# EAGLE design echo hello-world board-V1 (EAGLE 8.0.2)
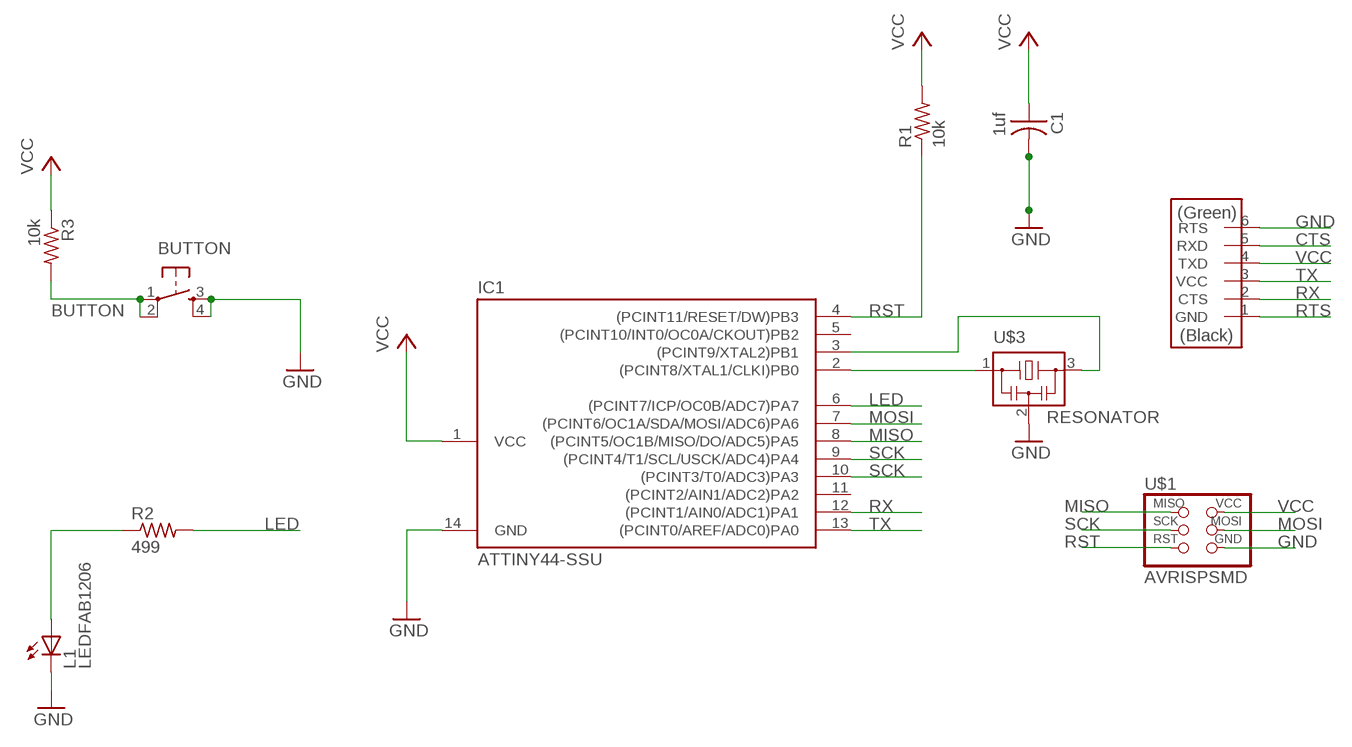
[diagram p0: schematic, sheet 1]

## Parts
BUTTON  6MM_SWITCH6MM_SWITCH  [6MM_SWITCH]
C1  1uf  CAP-US1206FAB  [C1206FAB]
IC1  ATTINY44-SSU  [SOIC14]
L1  LEDFAB1206  [LED1206FAB]
R1  10k  RES-US1206FAB  [R1206FAB]
R2  499  RES-US1206FAB  [R1206FAB]
R3  10k  RES-US1206FAB  [R1206FAB]
U$1  AVRISPSMD  [2X03SMD]
U$2  FTDI-SMD-HEADER  [1X06SMD]
U$3  RESONATOR  [EFOBM]

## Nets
BUTTON: BUTTON.1(P) BUTTON.2(P1) IC1.10((PCINT3/T0/ADC3)PA3) R3.2
CTS: U$2.5(RXD)
GND: BUTTON.3(S) BUTTON.4(S1) C1.2 IC1.14(GND) L1.2(C) U$1.6(GND) U$2.6(RTS) U$3.2
LED: IC1.6((PCINT7/ICP/OC0B/ADC7)PA7) R2.2
MISO: IC1.8((PCINT5/OC1B/MISO/DO/ADC5)PA5) U$1.1(MISO)
MOSI: IC1.7((PCINT6/OC1A/SDA/MOSI/ADC6)PA6) U$1.4(MOSI)
N$2: IC1.2((PCINT8/XTAL1/CLKI)PB0) U$3.1
N$3: IC1.3((PCINT9/XTAL2)PB1) U$3.3
N$6: L1.1(A) R2.1
RST: IC1.4((PCINT11/RESET/DW)PB3) R1.1 U$1.5(RST)
RTS: U$2.1(GND)
RX: IC1.12((PCINT1/AIN0/ADC1)PA1) U$2.2(CTS)
SCK: IC1.9((PCINT4/T1/SCL/USCK/ADC4)PA4) U$1.3(SCK)
TX: IC1.13((PCINT0/AREF/ADC0)PA0) U$2.3(VCC)
VCC: C1.1 IC1.1(VCC) R1.2 R3.1 U$1.2(VCC) U$2.4(TXD)
Unconnected: IC1.5((PCINT10/INT0/OC0A/CKOUT)PB2) IC1.11((PCINT2/AIN1/ADC2)PA2)

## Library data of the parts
BUTTON = 01_fab_2016:6MM_SWITCH: OMRON SWITCH
C1 = 01_fab_2016:CAP-US
IC1 = 01_fab_2016:ATTINY44
L1 = 01_fab_2016:LED: LED
R1-R3 = 01_fab_2016:RES-US: Resistor (US Symbol)
U$1 = 01_fab_2016:AVRISP
U$2 = 01_fab_2016:FTDI-SMD-HEADER
U$3 = 01_fab_2016:RESONATOR

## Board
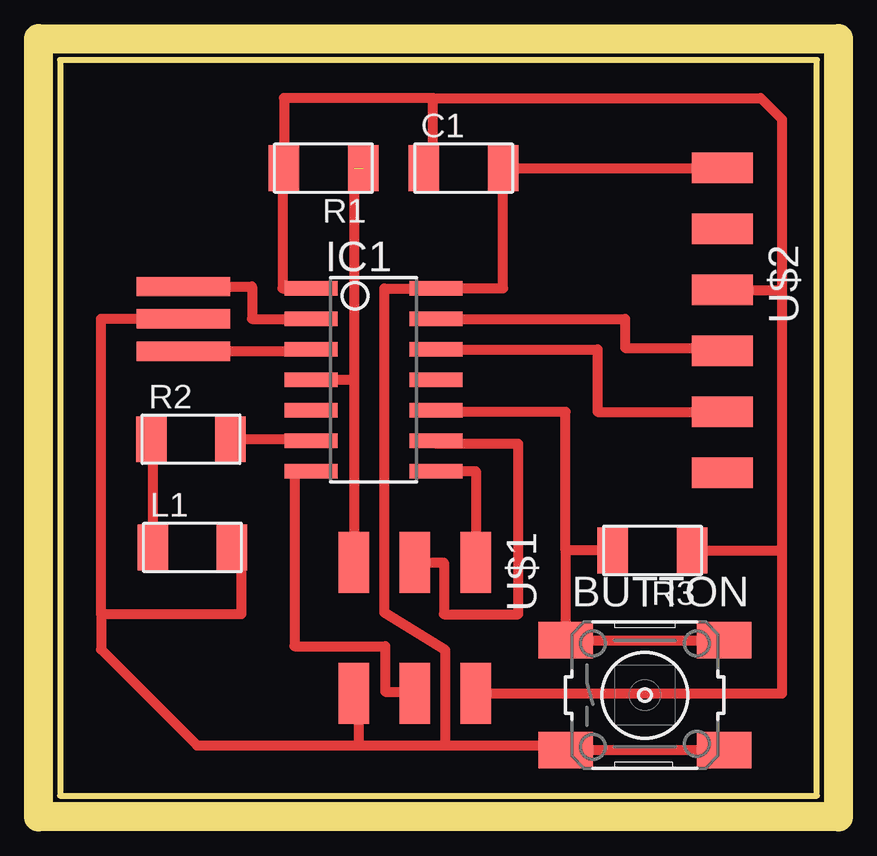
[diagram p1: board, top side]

Size 31.56 x 30.67 mm. Coordinates in mm from the lower left corner, seen from the top.
Outline: 0,0 31.56,0 31.56,30.67 0,30.67 0,0
Copper layers (1*16): Top 0.035mm / dielectric 1.5mm / Bottom 0.035mm
Design rules "default *": minimum track width 10mil, minimum drill 24mil, track to track 16mil, track to pad 16mil, pad to pad 16mil, via to via 16mil, smd to smd 16mil, copper to edge 40mil, drill to drill 8mil, minimum pad ring 10mil, minimum via ring 8mil, stop-mask expansion 4mil, vias tented up to drill 0mil, thermal gap 10mil
Milling: 4 lines

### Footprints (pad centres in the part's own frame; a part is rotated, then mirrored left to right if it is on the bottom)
6MM_SWITCH = smd 2.286 x 1.524: 1 -3.302,2.286; 2 3.302,2.286; 3 -3.302,-2.286; 4 3.302,-2.286
C1206FAB = smd 1.27 x 1.905: 1 -1.651,0; 2 1.651,0
SOIC14 = smd 0.61 x 2.21: 1 -3.81,-2.603; 2 -2.54,-2.603; 3 -1.27,-2.603; 4 0,-2.603; 5 1.27,-2.603; 6 2.54,-2.603; 7 3.81,-2.603; 8 3.81,2.603; 9 2.54,2.603; 10 1.27,2.603; 11 0,2.603; 12 -1.27,2.603; 13 -2.54,2.603; 14 -3.81,2.603
LED1206FAB = smd 1.27 x 1.905: 1 -1.651,0; 2 1.651,0
R1206FAB = smd 1.27 x 1.905: 1 -1.651,0; 2 1.651,0
2X03SMD = smd 2.54 x 1.27: 1 -2.54,2.54; 2 2.92,2.54; 3 -2.54,0; 4 2.92,0; 5 -2.54,-2.54; 6 2.92,-2.54
1X06SMD = smd 2.54 x 1.27: 1 0,6.35; 2 0,3.81; 3 0,1.27; 4 0,-1.27; 5 0,-3.81; 6 0,-6.35
EFOBM = smd 0.8 x 3.9: 1 -1.35,0; 2 0,0; 3 1.35,0

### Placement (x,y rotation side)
BUTTON  24.38,4.19 0 top
C1  16.83,26.16 0 top
IC1  13.08,17.34 270 top
L1  5.52,10.35 0 top
R1  10.99,26.16 180 top
R2  5.46,14.86 0 top
R3  24.7,10.22 180 top
U$1  14.8,7.18 270 top
U$2  27.62,19.81 180 top
U$3  5.14,19.88 270 top

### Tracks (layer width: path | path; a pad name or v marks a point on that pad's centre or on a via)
BUTTON
  Top 0.406: BUTTON.2 BUTTON.1 21.08,10.22 | R3.2 21.08,10.22 | 21.08,10.22 21.08,16 15.68,16 IC1.10
GND
  Top 0.406: U$2.6 C1.2 18.48,21.15 IC1.14 13.52,21.15 13.52,7.62 16.07,6.06 16.07,2.1 | U$3.2 1.71,19.88 1.71,7.56 | 1.71,7.56 1.71,6.1 5.72,2.1 12.45,2.1 | 12.45,2.1 16.07,2.1 | U$1.6 12.45,4.25 12.45,2.1 | L1.2 7.56,10.35 7.56,7.56 1.71,7.56 | 16.07,2.1 21.08,2.1 BUTTON.3 BUTTON.4
LED
  Top 0.406: R2.2 10.48,14.86 IC1.6
MISO
  Top 0.406: IC1.8 17.34,13.53 U$1.1
MOSI
  Top 0.406: IC1.7 9.78,13.53 9.78,6.22 13.56,6.22 13.56,4.33 14.8,4.33 U$1.4
N$2
  Top 0.406: U$3.1 8,21.23 8,19.88 IC1.2
N$3
  Top 0.406: U$3.3 10.48,18.53 IC1.3
N$6
  Top 0.406: R2.1 3.87,14.86 L1.1
RST  (1 unrouted)
  Top 0.406: 12.26,26.16 12.26,17.34 | 12.26,17.34 IC1.4 | 12.26,17.34 U$1.5
RX
  Top 0.406: IC1.12 22.41,18.61 22.41,16 U$2.2
SCK
  Top 0.406: U$1.3 16,9.71 16,7.56 19.11,7.56 19.11,14.67 15.68,14.67 IC1.9
TX
  Top 0.406: IC1.13 23.56,19.88 23.56,18.67 27.62,18.67 U$2.3
VCC
  Top 0.406: C1.1 15.56,26.16 15.56,29.08 | 15.56,29.08 9.33,29.08 R1.2 9.27,26.16 9.27,21.15 IC1.1 | U$1.2 30.1,4.25 30.1,10.22 | 30.1,21.08 30.1,10.22 | 30.1,21.08 30.1,28.19 29.21,29.08 15.56,29.08 | R3.1 30.1,10.22 | U$2.4 30.1,21.08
